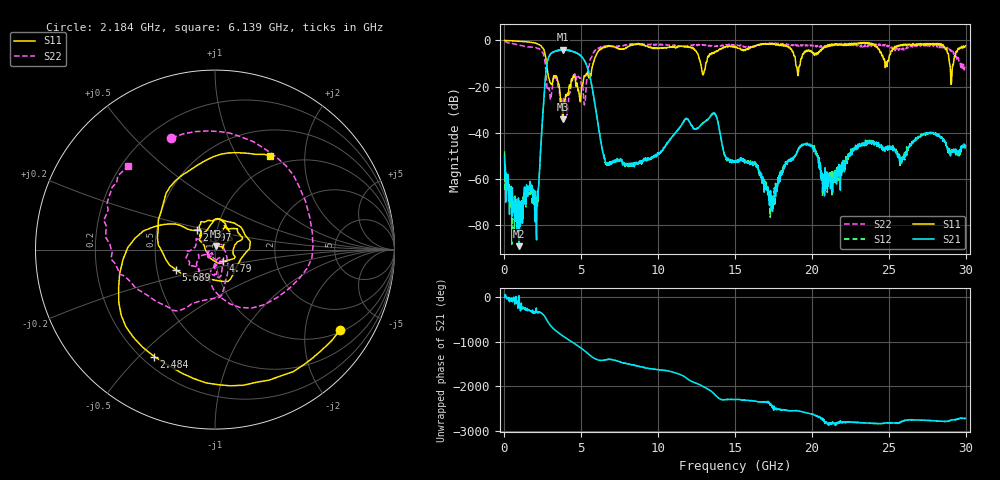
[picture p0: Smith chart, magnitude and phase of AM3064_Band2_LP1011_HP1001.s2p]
# Hz S DB R 50.0
!freq dBS11 angS11 dBS21 angS21 dBS12 angS12 dBS22 angS22
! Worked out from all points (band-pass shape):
!   1600 points, 10 MHz to 29.98 GHz, reference 50 ohm
!   highest |S21| = -4.04 dB at 3.815 GHz (marker M1); lowest = -89.1 dB at 965.9 MHz (marker M2)
!   |S21| within 3 dB of the highest: 2.894 GHz to 5.021 GHz (2.127 GHz wide, 53.7 % of centre)
!   lowest |S11| = -34.1 dB at 3.796 GHz (marker M3), VSWR 1.04, Z = 50.6 + j1.89 ohm
!   |S11| at or under -10 dB: 2.731 GHz to 5.764 GHz (3.032 GHz wide, 71.4 % of centre); 12.76 GHz to 13.1 GHz (334.6 MHz wide, 2.59 % of centre); 18.95 GHz to 19.24 GHz (294.4 MHz wide, 1.54 % of centre)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
!   |S22| runs from -32.3 to -0.3 dB; largest |S21 - S12| = 0.016
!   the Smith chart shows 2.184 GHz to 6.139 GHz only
!   S11 on the Smith chart (normalised r, x): 2.184 GHz: 1.08, -3.07; 2.484 GHz: 0.25, -0.55; 2.897 GHz: 0.80, +0.18; 4.79 GHz: 1.09, -0.14; 5.689 GHz: 0.63, -0.15; 6.139 GHz: 0.84, +1.39
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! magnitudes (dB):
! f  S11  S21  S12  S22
! 10 MHz  0.0  -50.1  -48.1  -0.3
! 965.9 MHz  -0.3  -89.1  -72.8  -2.0
! 2.184 GHz  -1.6  -68.7  -69.8  -3.5
! 2.484 GHz  -3.3  -33.2  -33.1  -5.3
! 2.897 GHz  -16.6  -7.0  -6.9  -20.6
! 3.796 GHz  -34.1  -4.1  -4.0  -27.8
! 3.815 GHz  -31.8  -4.0  -4.0  -26.3
! 4.79 GHz  -21.9  -5.7  -5.6  -15.7
! 5.015 GHz  -20.2  -7.0  -7.0  -19.1
! 5.689 GHz  -12.2  -19.9  -19.9  -6.9
! 6.139 GHz  -4.3  -38.7  -38.4  -3.5
! 6.702 GHz  -2.6  -54.1  -54.1  -2.5
! 10 GHz  -3.4  -48.9  -49.3  -1.9
! 13.6 GHz  -5.3  -31.8  -31.6  -2.5
! 15 GHz  -2.8  -52.8  -52.5  -1.9
! 17.39 GHz  -1.6  -70.8  -67.3  -1.3
! 19.99 GHz  -4.8  -46.0  -45.6  -2.0
! 21.21 GHz  -2.3  -64.3  -57.9  -2.1
! 25 GHz  -8.6  -46.2  -46.1  -2.3
! 28.28 GHz  -1.4  -41.1  -41.6  -3.2
! 29.08 GHz  -17.7  -48.2  -47.3  -5.1
! 29.98 GHz  -2.4  -45.9  -45.5  -10.3
